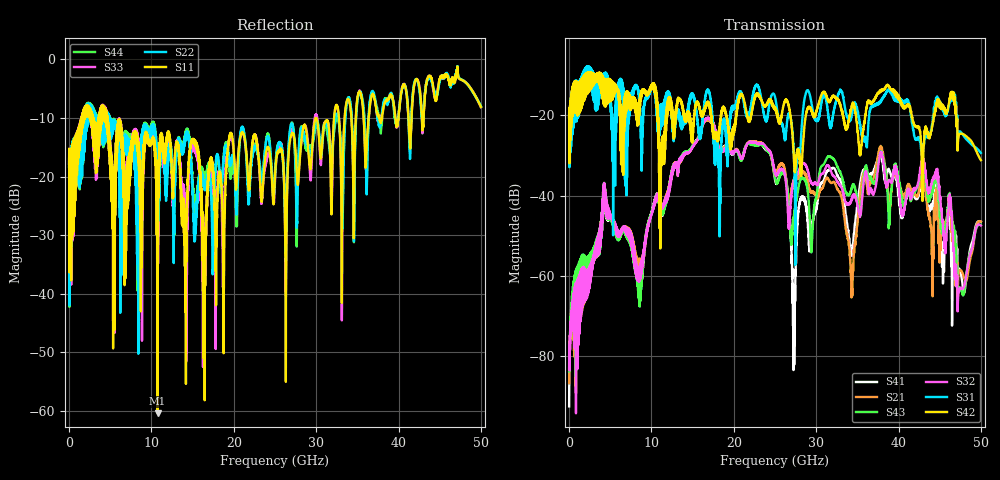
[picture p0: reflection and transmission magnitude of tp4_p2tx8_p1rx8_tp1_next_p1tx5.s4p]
! 100G CR Analysis
! File: tp4_p2tx8_p1rx8_tp1_next_p1tx5
! Description: 2m Cu Cable, OSFP, TP1-TP4
! Port Mapping
! Port1 -- P1RX8N
! Port2 -- P1TX5N
! Port3 -- P1RX8P
! Port4 -- P1TX5P
# GHz S MA R 50.00
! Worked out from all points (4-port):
!   5000 points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, 10 MHz to 50 GHz, reference 50 ohm
!   strongest paths, dB at 10 MHz, 12.51 GHz, 25.01 GHz, 37.51 GHz, 50 GHz:
!     S42: -20.5, -17.9, -18.0, -14.7, -31.2
!     S31: -20.6, -20.0, -15.5, -17.2, -29.4
!     S32: -83.1, -33.8, -34.4, -33.5, -47.5
!     S43: -83.7, -33.5, -35.5, -32.6, -47.3
!     S21: -86.7, -33.5, -35.0, -30.2, -46.5
!     S41: -92.4, -33.3, -36.1, -30.9, -46.5
!   lowest |S11| = -60.4 dB at 10.75 GHz (marker M1), VSWR 1.00, Z = 50.1 + j0.0204 ohm
!   |S11| at or under -10 dB: start of sweep to 1.499 GHz; 4.65 GHz to 32.18 GHz (27.53 GHz wide, 149 % of centre); 32.77 GHz to 33.46 GHz (688 MHz wide, 2.08 % of centre)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
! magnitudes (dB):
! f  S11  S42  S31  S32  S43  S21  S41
! 10 MHz  -17.8  -20.5  -20.6  -83.1  -83.7  -86.7  -92.4
! 4.28 GHz  -10.5  -11.8  -11.5  -41.8  -41.8  -41.7  -42.0
! 10.75 GHz  -60.4  -19.1  -20.5  -39.5  -39.5  -39.5  -39.4
! 23.38 GHz  -24.1  -16.5  -16.5  -27.0  -27.2  -26.9  -27.2
! 27.31 GHz  -13.1  -31.6  -30.9  -35.9  -44.5  -35.9  -70.7
! 31.91 GHz  -21.5  -15.5  -21.6  -34.6  -30.6  -36.8  -33.2
! 50 GHz  -8.1  -31.2  -29.4  -47.5  -47.3  -46.5  -46.5
